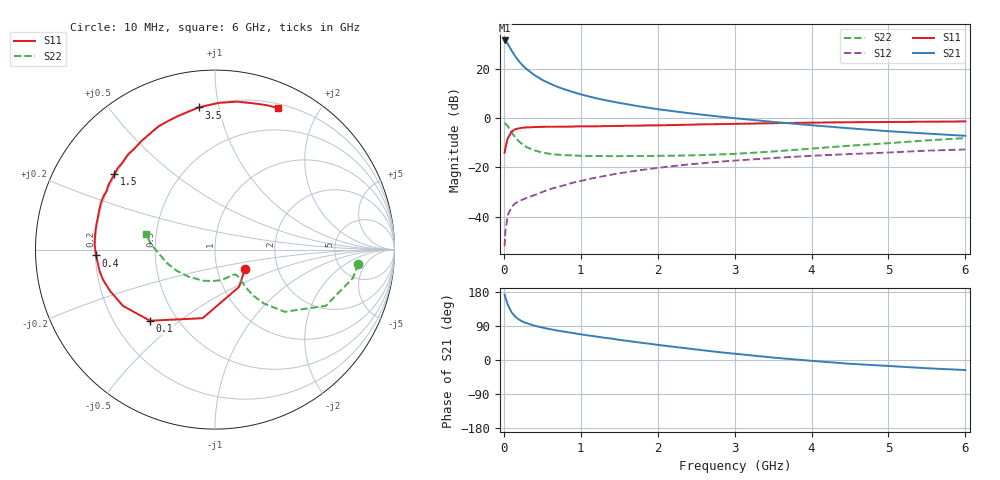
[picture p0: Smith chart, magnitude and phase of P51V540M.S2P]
! SIEMENS Small Signal Semiconductors
! BFP183
! Si NPN RF Bipolar Junction Transistor in SOT143
! VCE = 1.5 V  IC = 40 mA
! Common Emitter S-Parameters:  March  1996
# GHz  S  MA  R  50
!  f  S11  S21  S12  S22
! GHz  MAG  ANG  MAG  ANG  MAG  ANG  MAG  ANG
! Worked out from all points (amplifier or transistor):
!   36 points, 10 MHz to 6 GHz, reference 50 ohm
!   highest |S21| = 31.7 dB at 10 MHz (marker M1)
!   |S21| within 3 dB of that: start of sweep to 80.63 MHz
!   unconditionally stable (mu >= 1): start of sweep to 18.65 MHz; 265.8 MHz to end of sweep
!   at 250 MHz: K = 0.97, MSG = 27.2 dB, |S12| = -33.0 dB
!   at 1.4 GHz: K = 1.56, MAG = 10.5 dB, |S12| = -22.9 dB
!   at 6 GHz: K = 1.23, MAG = -0.1 dB, |S12| = -12.7 dB
!   S11 on the Smith chart (normalised r, x): 10 MHz: 1.36, -0.31; 100 MHz: 0.35, -0.39; 400 MHz: 0.20, -0.02; 1.5 GHz: 0.19, +0.32; 3.5 GHz: 0.20, +0.87; 6 GHz: 0.24, +1.52
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0.01  0.1995 -32.6  38.49 172.7  0.0025 72.9  0.8022 -5.7
0.02  0.2473 -57.3  37.81 165.7  0.005 72.0  0.784 -11.7
0.05  0.3882 -100.2  33.15 146.6  0.0106 65.0  0.6924 -26.9
0.1  0.5367 -132.4  24.07 125.9  0.0158 49.7  0.5199 -41.8
0.15  0.6008 -148.5  18.16 113.9  0.0186 46.0  0.4051 -47.8
0.2  0.6278 -158.3  14.3 106.3  0.0209 46.5  0.3346 -50.2
0.25  0.646 -164.8  11.69 100.7  0.0223 47.2  0.2891 -50.7
0.3  0.654 -169.4  9.913 96.9  0.0242 48.7  0.2571 -50.5
0.4  0.6637 -177.2  7.551 90.4  0.0275 51.5  0.2222 -49.8
0.5  0.6719 177.4  6.054 85.6  0.0317 53.3  0.2017 -49.4
0.6  0.6736 172.4  5.097 81.3  0.0363 56.0  0.1895 -49.7
0.7  0.6754 168.3  4.353 77.6  0.0399 57.2  0.1822 -50.2
0.9  0.6812 161.6  3.427 71.2  0.0491 58.1  0.1757 -52.8
1.1  0.6884 154.3  2.802 64.7  0.0581 58.9  0.1714 -56.5
1.5  0.7009 143.1  2.063 53.2  0.0764 57.6  0.17 -66.4
1.8  0.7129 134.4  1.718 45.2  0.0893 55.3  0.1709 -75.3
2.2  0.7304 124.3  1.4 35.0  0.1066 51.5  0.1734 -88.3
2.8  0.7622 110.2  1.087 20.7  0.1307 45.3  0.1843 -109.8
3.5  0.7972 96.6  0.846 6.4  0.1558 38.3  0.2115 -134.7
4.5  0.8334 81.5  0.626 -10.0  0.1875 28.2  0.2778 -164.3
5.5  0.8538 70.6  0.49 -21.8  0.2198 19.0  0.3562 175.5
6  0.8642 65.9  0.441 -26.5  0.2325 13.9  0.396 167.1
